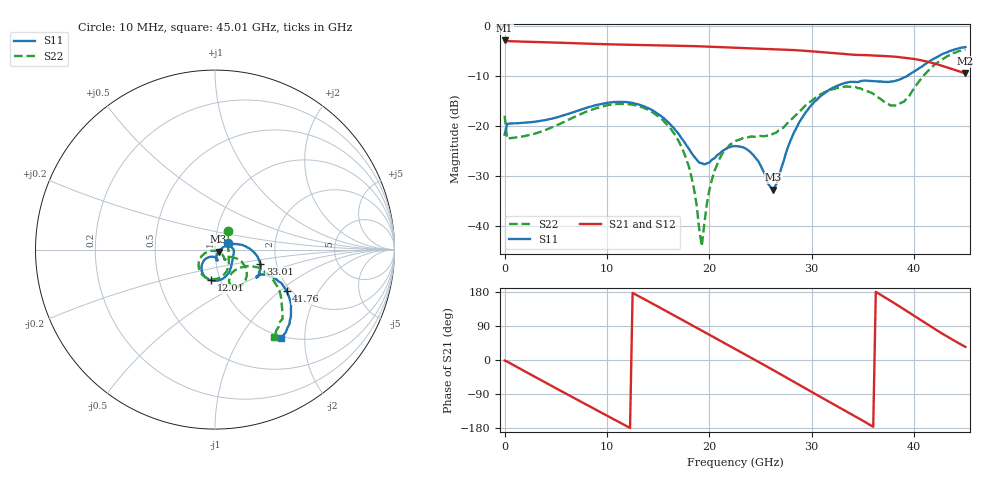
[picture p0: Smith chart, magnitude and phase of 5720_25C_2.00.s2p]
! Device:  ADRF5720
! Description: 0.5dB LSB GaAs MMIC 6-bit Digital Attenuator
! Frequency:  0.000009 -  40 GHz
! Ports:
!	RF1	= Port 1
!	RF2	= Port 2
! Vdd:  3.3 Volt
! Vss:  -3.3 Volt
! Control:  0/3.3 Volt
! State:  2.00 dB attenuation
! Data:  The device was measured using G-S-G Probes on a matrix board.
!  Data was collected using an calibrated 4 port network analyzer.
!  The reference plane for this measurement is at the launchers.
! Note:  Analog Devices supplies this data as a sample of measured data
!  for this product.  Your particular data for this product may vary.
!  Data was taken at 25 degrees C.
!  Analog Devices reserves the right to change this data at anytime.
# GHZ S DB R 45.0
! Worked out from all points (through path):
!   181 points, 10 MHz to 45.01 GHz, reference 45 ohm
!   highest |S21| = -2.87 dB at 10 MHz (marker M1); lowest = -9.5 dB at 45.01 GHz (marker M2)
!   group delay of S21, straight-line fit = 42 ps
!   lowest |S11| = -32.8 dB at 26.26 GHz (marker M3), VSWR 1.05, Z = 46.8 - j1.05 ohm
!   |S11| at or under -10 dB: start of sweep to 39.32 GHz
!   |S22| runs from -44.1 to -4.6 dB; largest |S21 - S12| = 0.00082
!   S11 on the Smith chart (normalised r, x): 10 MHz: 1.15, +0.08; 12.01 GHz: 0.90, -0.32; 33.01 GHz: 1.65, -0.28; 41.76 GHz: 1.90, -1.12; 45.01 GHz: 0.96, -1.54
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0.01  -21.77 26.4  -2.87 -1.4  -2.87 -1.4  -17.96 56.5
0.26  -19.61 -0.2  -3.00 -4.2  -3.00 -4.2  -22.64 0.7
4.26  -18.72 -34.2  -3.25 -63.3  -3.25 -63.3  -20.63 -34.4
7.76  -16.54 -58.5  -3.48 -114.4  -3.48 -114.4  -17.35 -61.3
12.01  -15.26 -97.6  -3.73 -175.7  -3.73 -175.7  -15.63 -104.0
15.26  -17.99 -126.8  -3.84 136.9  -3.84 137.0  -18.49 -140.0
18.01  -24.59 -131.6  -3.98 96.3  -3.97 96.3  -28.21 -165.0
18.76  -26.76 -119.7  -4.02 85.1  -4.02 85.2  -35.85 -155.6
19.26  -27.50 -107.5  -4.06 77.7  -4.06 77.7  -44.14 -100.7
19.76  -27.55 -94.6  -4.09 70.3  -4.09 70.3  -35.67 -37.0
20.51  -26.50 -82.5  -4.15 59.1  -4.15 59.1  -29.02 -29.8
22.76  -24.09 -78.9  -4.33 25.7  -4.33 25.7  -22.89 -43.0
24.26  -25.76 -82.9  -4.45 3.3  -4.45 3.3  -22.16 -46.5
26.26  -32.78 -29.3  -4.60 -26.9  -4.60 -26.8  -21.54 -33.7
28.26  -21.40 18.9  -4.80 -57.5  -4.81 -57.4  -18.22 -22.6
30.26  -15.21 5.8  -5.09 -88.3  -5.09 -88.2  -14.53 -28.5
33.01  -11.55 -17.4  -5.55 -130.2  -5.55 -130.2  -12.26 -48.4
35.51  -10.97 -32.1  -5.83 -168.4  -5.84 -168.4  -13.11 -64.7
37.76  -11.11 -31.7  -6.07 155.2  -6.08 155.3  -15.96 -53.5
40.01  -9.07 -25.5  -6.59 116.7  -6.59 116.8  -12.42 -23.6
41.76  -6.72 -30.2  -7.36 86.3  -7.36 86.4  -8.21 -29.4
45.01  -4.19 -53.2  -9.46 34.6  -9.46 34.7  -4.65 -56.0
